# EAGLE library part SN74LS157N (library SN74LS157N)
Quadruple 2-Line To 1-Line Data Selectors/Multiplexers Source: Datasheet
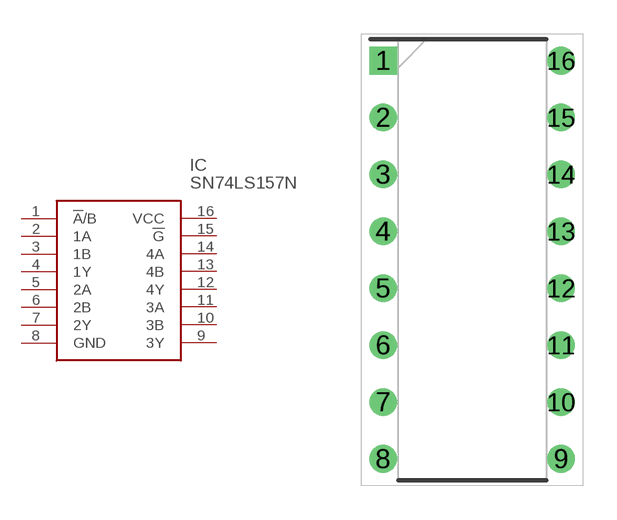
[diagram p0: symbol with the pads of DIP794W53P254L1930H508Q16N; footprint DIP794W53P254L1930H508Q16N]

Designator prefix IC

## SN74LS157N (Arrow_Part_Number: SN74LS157N; Arrow_Price-Stock: https://www.arrow.com/en/products/sn74ls157n/texas-instruments?region=nac; Description: Quadruple 2-Line To 1-Line Data Selectors/Multiplexers; Height: 5.08mm; Manufacturer_Name: Texas Instruments; Manufacturer_Part_Number: SN74LS157N; Mouser_Part_Number: 595-SN74LS157N; Mouser_Price-Stock: https://www.mouser.co.uk/ProductDetail/Texas-Instruments/SN74LS157N?qs=LzFo6vGRJ4stINDkpW5nIA%3D%3D)  [DIP794W53P254L1930H508Q16N]
1  !A!/B
2  1A
3  1B
4  1Y
5  2A
6  2B
7  2Y
8  GND
9  3Y
10  3B
11  3A
12  4Y
13  4B
14  4A
15  !G
16  VCC

## Footprint DIP794W53P254L1930H508Q16N (pad centres in mm)
16 pdip
drill 0.73 pad 1.13 square: 1 -3.97,8.89
drill 0.73 pad 1.13: 2 -3.97,6.35; 3 -3.97,3.81; 4 -3.97,1.27; 5 -3.97,-1.27; 6 -3.97,-3.81; 7 -3.97,-6.35; 8 -3.97,-8.89; 9 3.97,-8.89; 10 3.97,-6.35; 11 3.97,-3.81; 12 3.97,-1.27; 13 3.97,1.27; 14 3.97,3.81; 15 3.97,6.35; 16 3.97,8.89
